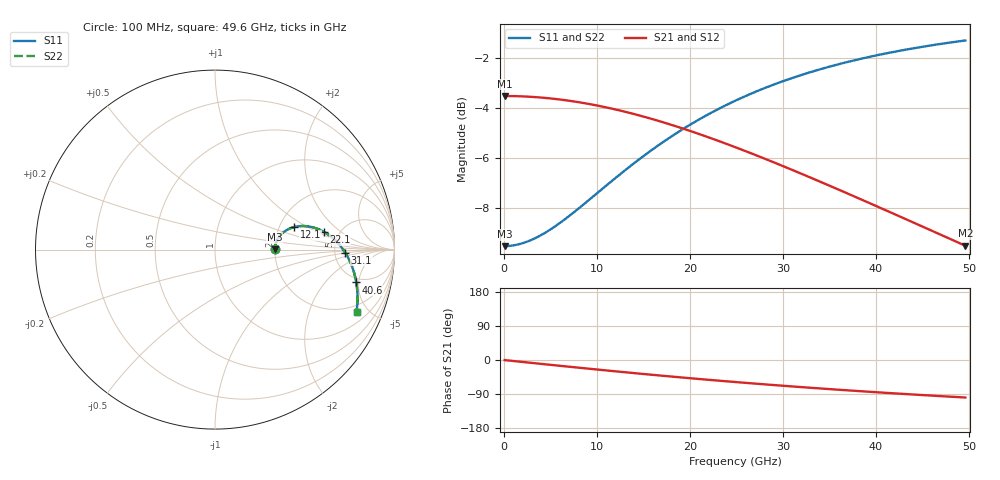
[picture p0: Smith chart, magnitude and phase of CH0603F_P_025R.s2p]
# GHz S RI R 25
! S-Parameters data
! Freq  reS11  imS11  reS21  imS21  reS12  imS12  reS22  imS22
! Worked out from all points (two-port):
!   100 points, 100 MHz to 49.6 GHz, reference 25 ohm
!   highest |S21| = -3.52 dB at 100 MHz (marker M1); lowest = -9.5 dB at 49.6 GHz (marker M2)
!   |S21| within 3 dB of the highest: start of sweep to 31.23 GHz
!   lowest |S11| = -9.5 dB at 100 MHz (marker M3), VSWR 2.00, Z = 50 + j0.156 ohm
!   |S11| at or under -10 dB: nowhere
!   |S22| runs from -9.5 to -1.3 dB; largest |S21 - S12| = 0
!   S11 on the Smith chart (normalised r, x): 100 MHz: 2.00, +0.01; 12.1 GHz: 2.40, +0.76; 22.1 GHz: 3.78, +1.20; 31.1 GHz: 6.25, -0.44; 40.6 GHz: 4.40, -4.64; 49.6 GHz: 1.57, -4.21
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0.1  0.3333 0.00139  0.6667 -0.00296  0.6667 -0.00296  0.3333 0.00139
1.6  0.3355 0.0221  0.6642 -0.0472  0.6642 -0.0472  0.3355 0.0221
3.6  0.344 0.0488  0.6544 -0.1053  0.6544 -0.1053  0.344 0.0488
6.1  0.3633 0.0788  0.6321 -0.1744  0.6321 -0.1744  0.3633 0.0788
8.6  0.391 0.1033  0.5999 -0.2378  0.5999 -0.2378  0.391 0.1033
10.6  0.418 0.1178  0.5682 -0.2832  0.5682 -0.2832  0.418 0.1178
12.1  0.4405 0.1254  0.5416 -0.3137  0.5416 -0.3137  0.4405 0.1254
14.6  0.4808 0.1312  0.4932 -0.3576  0.4932 -0.3576  0.4808 0.1312
16.6  0.5145 0.1298  0.452 -0.3862  0.452 -0.3862  0.5145 0.1298
19.1  0.557 0.1204  0.399 -0.4139  0.399 -0.4139  0.557 0.1204
20.6  0.5819 0.1111  0.367 -0.4264  0.367 -0.4264  0.5819 0.1111
22.1  0.6062 0.099  0.3353 -0.436  0.3353 -0.436  0.6062 0.099
25.1  0.6516 0.0679  0.2736 -0.4474  0.2736 -0.4474  0.6516 0.0679
28.1  0.6916 0.0288  0.2155 -0.4497  0.2155 -0.4497  0.6916 0.0288
31.1  0.7252 -0.0166  0.1622 -0.4444  0.1622 -0.4444  0.7252 -0.0166
33.1  0.7439 -0.0495  0.1295 -0.4376  0.1295 -0.4376  0.7439 -0.0495
36.6  0.7693 -0.1104  0.0781 -0.4206  0.0781 -0.4206  0.7693 -0.1104
38.6  0.7796 -0.1465  0.052 -0.4088  0.052 -0.4088  0.7796 -0.1465
40.6  0.7871 -0.1831  0.0283 -0.3958  0.0283 -0.3958  0.7871 -0.1831
41.6  0.7898 -0.2015  0.0173 -0.3889  0.0173 -0.3889  0.7898 -0.2015
45.6  0.794 -0.2748  -0.0213 -0.36  -0.0213 -0.36  0.794 -0.2748
49.6  0.7886 -0.3466  -0.0522 -0.3299  -0.0522 -0.3299  0.7886 -0.3466
